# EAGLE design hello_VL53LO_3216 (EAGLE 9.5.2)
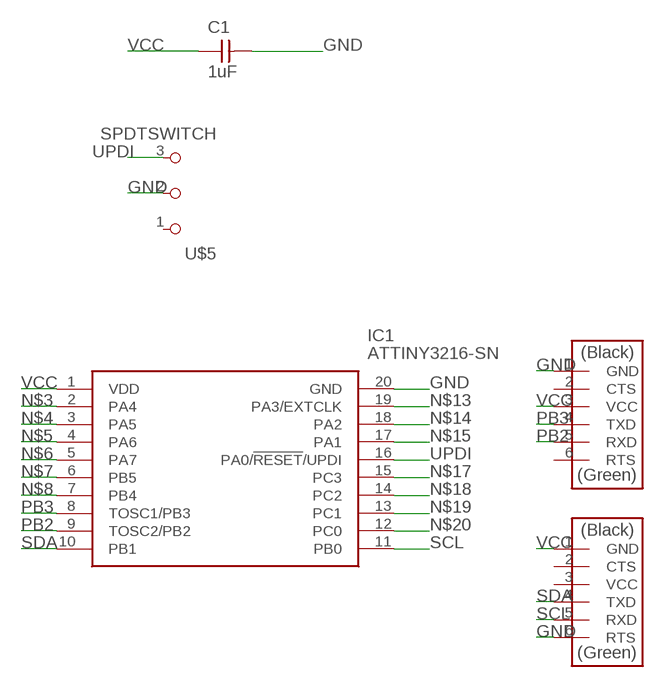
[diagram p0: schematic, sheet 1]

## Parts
C1  1uF  CAP_UNPOLARIZEDFAB  [C1206FAB]
IC1  ATTINY3216-SN  [SOIC127P1030X265-20N]
U$1  CONN_06_FTDI-SMD-HEADER  [1X06SMD]
U$2  CONN_06_FTDI-SMD-HEADER  [1X06SMD]
U$5  SPDTSWITCH  [SPDTSWITCH]

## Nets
GND: C1.2 IC1.20(GND) U$1.6(RTS) U$2.1(GND) U$5.2
N$3: IC1.2(PA4)
N$4: IC1.3(PA5)
N$5: IC1.4(PA6)
N$6: IC1.5(PA7)
N$7: IC1.6(PB5)
N$8: IC1.7(PB4)
N$13: IC1.19(PA3/EXTCLK)
N$14: IC1.18(PA2)
N$15: IC1.17(PA1)
N$17: IC1.15(PC3)
N$18: IC1.14(PC2)
N$19: IC1.13(PC1)
N$20: IC1.12(PC0)
PB2: IC1.9(TOSC2/PB2) U$2.5(RXD)
PB3: IC1.8(TOSC1/PB3) U$2.4(TXD)
SCL: IC1.11(PB0) U$1.5(RXD)
SDA: IC1.10(PB1) U$1.4(TXD)
UPDI: IC1.16(PA0/!RESET!/UPDI) U$5.3
VCC [New Class]: C1.1 IC1.1(VDD) U$1.1(GND) U$2.3(VCC)
Unconnected: U$1.2(CTS) U$1.3(VCC) U$2.2(CTS) U$2.6(RTS) U$5.1

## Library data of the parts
C1 = fab:CAP_UNPOLARIZED
IC1 = ATTINY3216-SN:ATTINY3216-SN: MICROCHIP - ATTINY3216-SN - 8 Bit MCU, AVR Family ATtiny3216 Series Microcontrollers, 20 MHz, 32 KB, 2 KB, 20 Pins, SOIC Source: Datasheet; AVAILABILITY: Unavailable; DESCRIPTION: AVR tinyAVR™ 1 Microcontroller IC 8-Bit 20MHz 32KB _32K x 8_ FLASH 20-SOIC; MF: Microchip Technology; MP: ATTINY3216-SN; PACKAGE: SOIC-20 Microchip Technology; PRICE: None
U$1 U$2 = fab:CONN_06_FTDI-SMD-HEADER
U$5 = fab:SPDTSWITCH

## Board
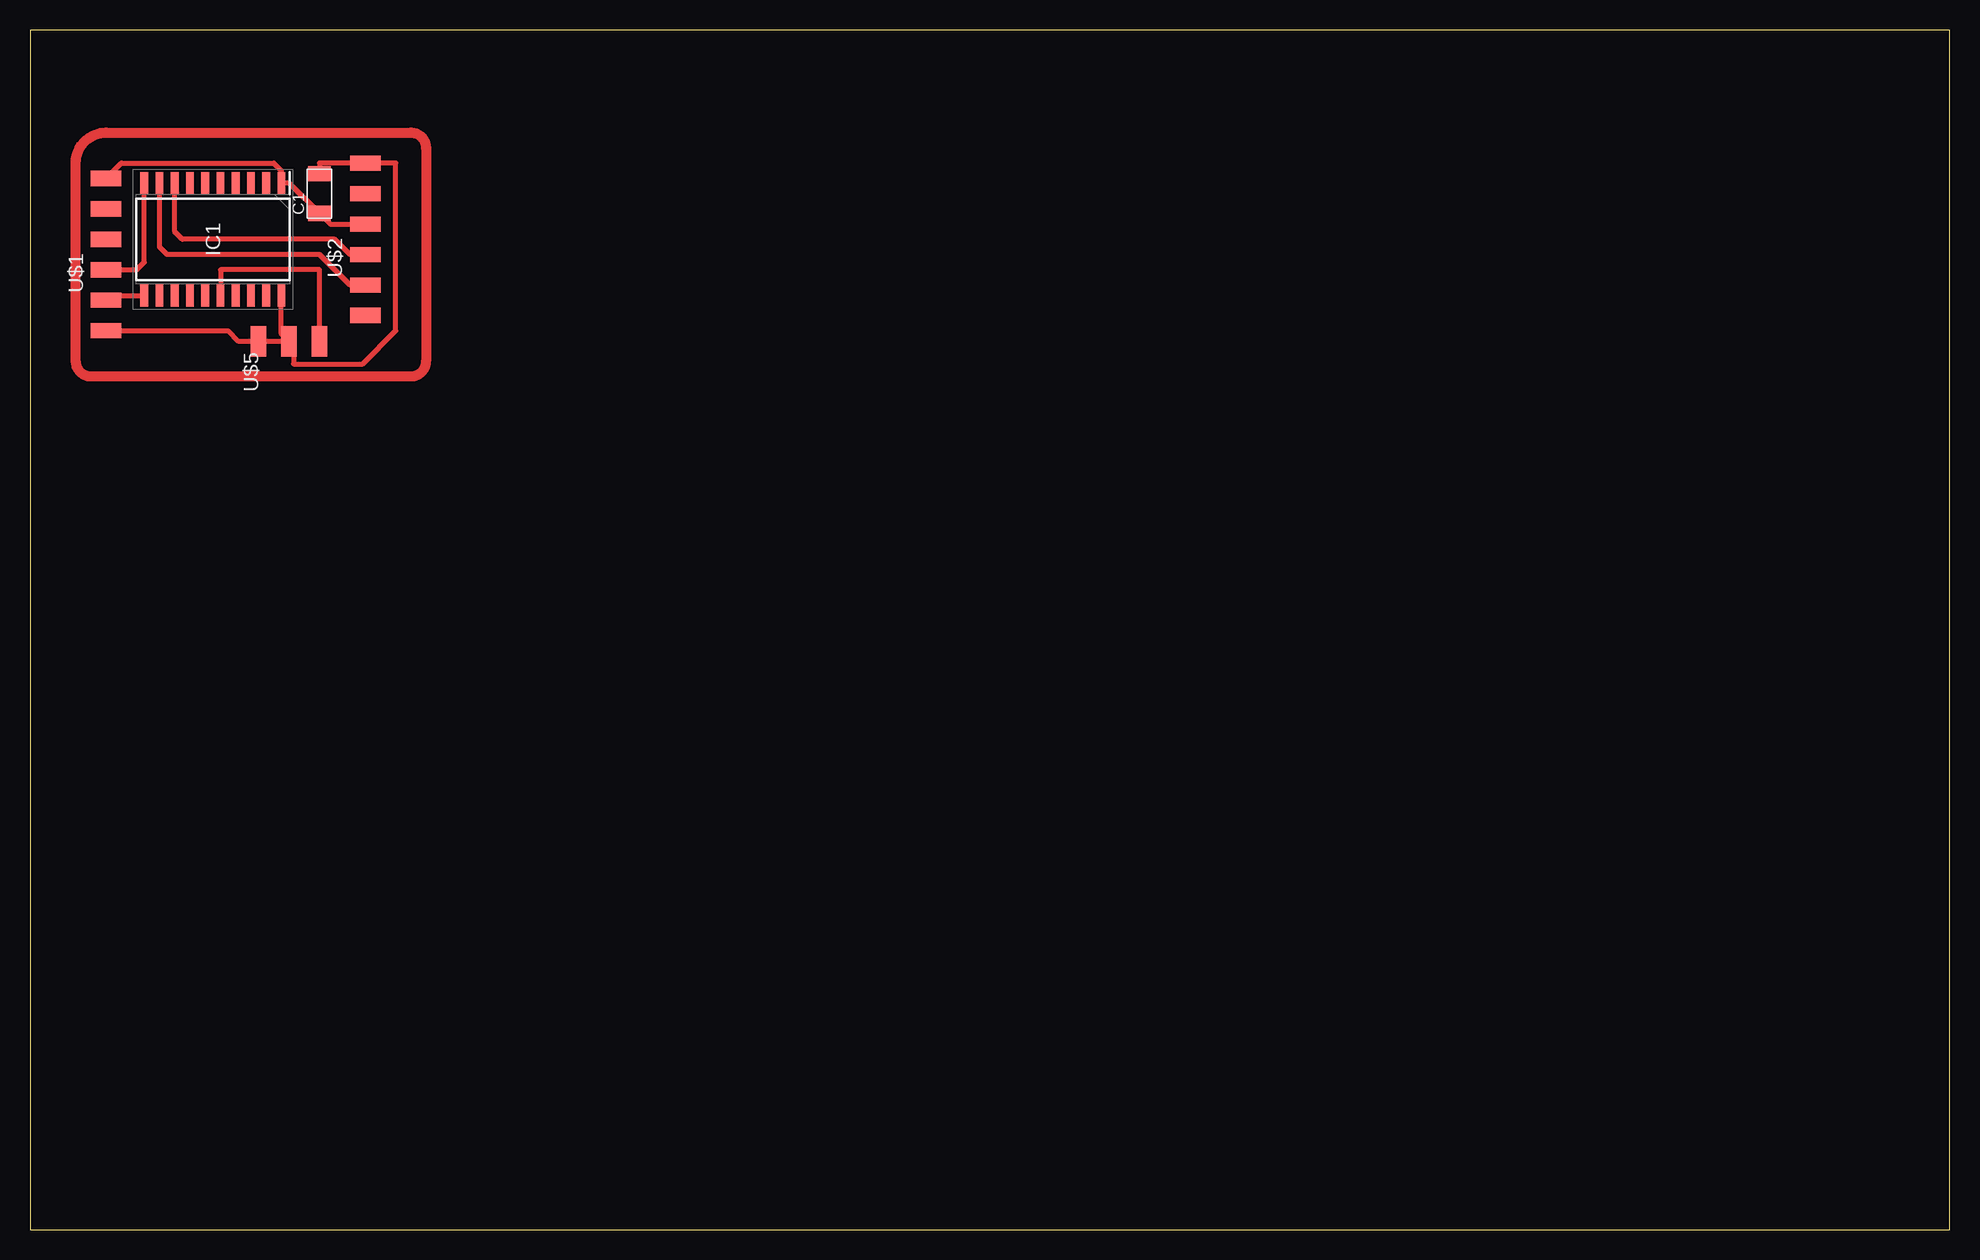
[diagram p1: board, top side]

Size 160 x 100 mm. Coordinates in mm from the lower left corner, seen from the top.
Outline: 0,0 160,0 160,100 0,100 0,0
Copper layers (1*16): Top 0.035mm / dielectric 1.5mm / Bottom 0.035mm
Design rules "default *": minimum track width 16mil, minimum drill 0.35mm, track to track 16mil, track to pad 16mil, pad to pad 16mil, via to via 16mil, smd to smd 16mil, copper to edge 40mil, drill to drill 6mil, minimum pad ring 10mil, minimum via ring 8mil, stop-mask expansion 4mil, vias tented up to drill 0mil, thermal gap 10mil

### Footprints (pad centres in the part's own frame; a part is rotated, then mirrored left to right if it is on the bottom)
C1206FAB = smd 1.27 x 1.905: 1 -1.651,0; 2 1.651,0
SOIC127P1030X265-20N = smd 1.85 x 0.65: 1 -4.675,5.715; 2 -4.675,4.445; 3 -4.675,3.175; 4 -4.675,1.905; 5 -4.675,0.635; 6 -4.675,-0.635; 7 -4.675,-1.905; 8 -4.675,-3.175; 9 -4.675,-4.445; 10 -4.675,-5.715; 11 4.675,-5.715; 12 4.675,-4.445; 13 4.675,-3.175; 14 4.675,-1.905; 15 4.675,-0.635; 16 4.675,0.635; 17 4.675,1.905; 18 4.675,3.175; 19 4.675,4.445; 20 4.675,5.715
1X06SMD = smd 2.54 x 1.27: 1 0,6.35; 2 0,3.81; 3 0,1.27; 4 0,-1.27; 5 0,-3.81; 6 0,-6.35
SPDTSWITCH = smd 2.54 x 1.27: 1 0.38,2.54; 2 0.38,0; 3 0.38,-2.54

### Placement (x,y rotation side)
C1  24.13,86.36 90 top
IC1  15.24,82.55 270 top
U$1  6.35,81.28 0 top
U$2  27.94,82.55 0 top
U$5  21.59,73.66 90 top

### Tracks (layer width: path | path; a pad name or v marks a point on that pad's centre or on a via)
GND
  Top 0.406: U$1.6 16.51,74.93 17.4,74.04 U$5.2 | U$5.2 21.59,73.66 | C1.2 24.13,88.9 U$2.1 30.48,88.9 30.48,74.93 27.71,72.16 21.97,72.16 21.97,73.66 U$5.2 | U$5.2 20.95,74.67 IC1.20
N$1
  Top 0.813: 6.35,91.44 31.75,91.44 arc-90 33.02,90.17 33.02,72.39 arc-90 31.75,71.12 5.08,71.12 arc-90 3.81,72.39 3.81,88.9 arc-90 6.35,91.44
PB2
  Top 0.406: U$2.5 26.67,78.74 24.13,81.28 11.43,81.28 10.79,81.92 IC1.9
PB3
  Top 0.406: U$2.4 26.67,81.28 25.4,82.55 12.7,82.55 12.06,83.19 IC1.8
SCL
  Top 0.406: U$1.5 6.75,77.88 IC1.11
SDA
  Top 0.406: U$1.4 8.89,80.01 9.53,80.64 IC1.10
UPDI
  Top 0.406: U$5.3 24.13,80.01 15.88,80.01 IC1.16
VCC
  Top 0.406: U$2.3 25.02,83.82 C1.1 21.61,87.22 IC1.1 20.95,88.27 20.32,88.9 7.62,88.9 U$1.1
